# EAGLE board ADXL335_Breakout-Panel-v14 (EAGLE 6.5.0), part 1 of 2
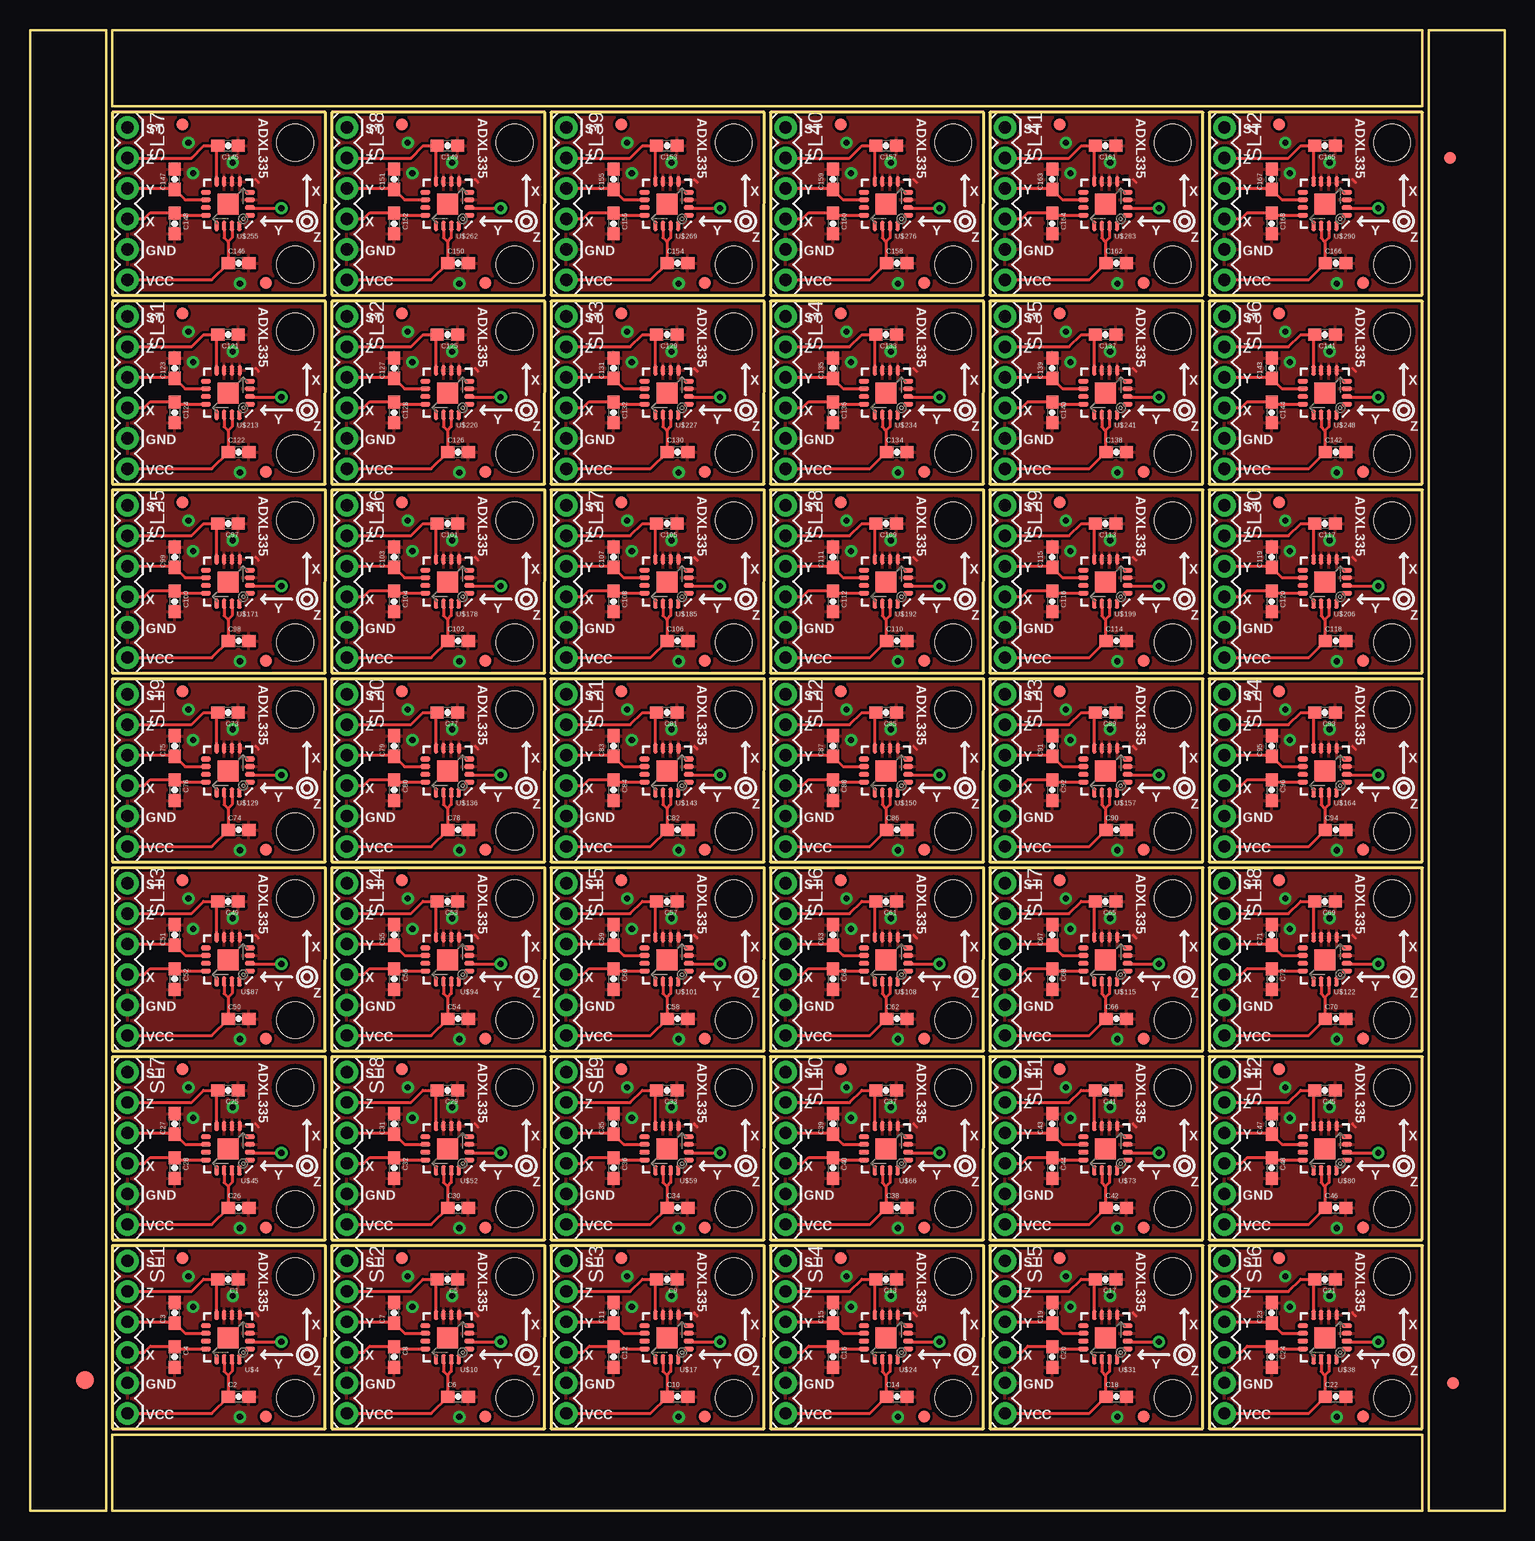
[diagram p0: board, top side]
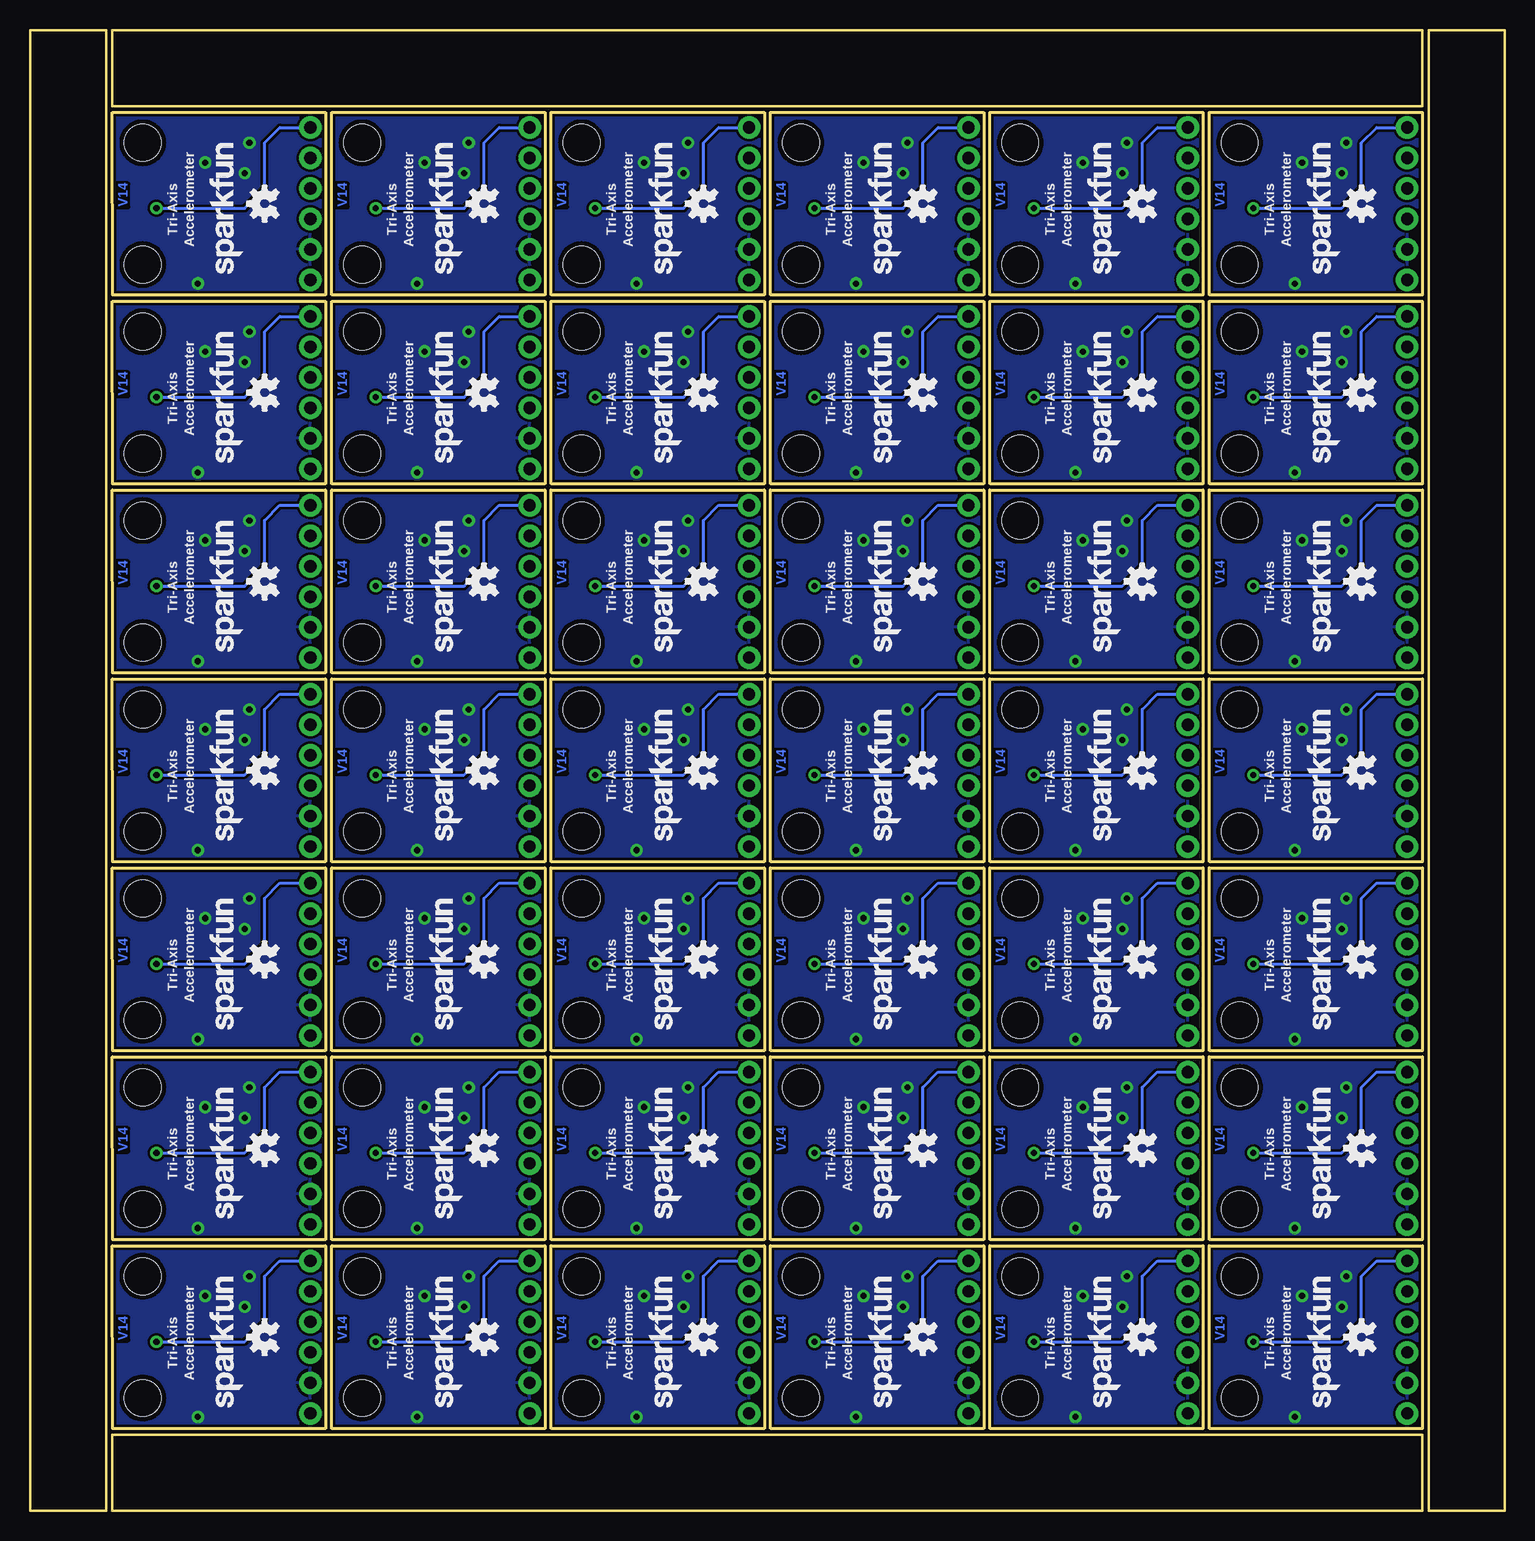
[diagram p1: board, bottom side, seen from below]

Size 122.94 x 123.44 mm. Coordinates in mm from the lower left corner, seen from the top.
Outline: 188 segments
Copper layers (1*16): Top 0.035mm / dielectric 1.5mm / Bottom 0.035mm
Design rules "SparkFun": minimum track width 7mil, minimum drill 15mil, track to track 8mil, track to pad 8mil, pad to pad 8mil, via to via 8mil, smd to smd 8mil, copper to edge 8mil, drill to drill 8mil, minimum pad ring 12mil, minimum via ring 10mil, stop-mask expansion 4mil, vias tented up to drill 20mil, thermal gap 10mil
tRestrict: area 16.4,16.3 to 16.6,16.4; area 17,16.3 to 17.3,16.4; area 18,15.7 to 18.4,16.9; area 34.7,16.3 to 34.9,16.4; area 35.3,16.3 to 35.6,16.4; area 36.3,15.7 to 36.7,16.9; area 53,16.3 to 53.2,16.4; area 53.6,16.3 to 53.9,16.4; area 54.6,15.7 to 55,16.9; area 71.2,16.3 to 71.5,16.4; area 71.9,16.3 to 72.2,16.4; area 72.9,15.7 to 73.3,16.9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

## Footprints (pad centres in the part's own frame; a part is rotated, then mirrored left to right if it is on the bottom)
0603-CAP = smd 1.1 x 1: 1 -0.85,0; 2 0.85,0
FIDUCIAL-1.5X3 = smd 1.5 x 1.5: 1 0,0
FIDUCIAL-1X2 = smd 1 x 1: 1 0,0
1X06 = drill 1.016 pad 1.88: 1 0,0; 2 2.54,0; 3 5.08,0; 4 7.62,0; 5 10.16,0; 6 12.7,0
ADXL335-P = smd 1.75 x 1.75: 0 0,0.051 | smd 0.838 x 0.37: 1 -1.826,0.975; 2 -1.826,0.325; 3 -1.826,-0.325; 4 -1.826,-0.95; 9 1.852,-0.95; 10 1.852,-0.325; 11 1.852,0.325; 12 1.852,0.975 | smd 0.37 x 0.838: 5 -0.975,-1.852; 6 -0.325,-1.852; 7 0.325,-1.852; 8 0.95,-1.852; 13 0.95,1.852; 14 0.325,1.852; 15 -0.325,1.852; 16 -0.95,1.852
STAND-OFF-TIGHT = hole 3.048: 0,0

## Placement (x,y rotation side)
C1  0.1uF  [0603-CAP]  16.51,19.3 180 top
C2  0.1uF  [0603-CAP]  17.4,9.53 0 top
C3  0.1uF  [0603-CAP]  12.06,16.51 90 top
C4  0.1uF  [0603-CAP]  12.06,12.83 270 top
C5  0.1uF  [0603-CAP]  34.8,19.3 180 top
C6  0.1uF  [0603-CAP]  35.69,9.53 0 top
C7  0.1uF  [0603-CAP]  30.35,16.51 90 top
C8  0.1uF  [0603-CAP]  30.35,12.83 270 top
C9  0.1uF  [0603-CAP]  53.09,19.3 180 top
C10  0.1uF  [0603-CAP]  53.98,9.53 0 top
C11  0.1uF  [0603-CAP]  48.64,16.51 90 top
C12  0.1uF  [0603-CAP]  48.64,12.83 270 top
C13  0.1uF  [0603-CAP]  71.37,19.3 180 top
C14  0.1uF  [0603-CAP]  72.26,9.53 0 top
C15  0.1uF  [0603-CAP]  66.93,16.51 90 top
C16  0.1uF  [0603-CAP]  66.93,12.83 270 top
C17  0.1uF  [0603-CAP]  89.66,19.3 180 top
C18  0.1uF  [0603-CAP]  90.55,9.53 0 top
C19  0.1uF  [0603-CAP]  85.22,16.51 90 top
C20  0.1uF  [0603-CAP]  85.22,12.83 270 top
C21  0.1uF  [0603-CAP]  107.95,19.3 180 top
C22  0.1uF  [0603-CAP]  108.84,9.53 0 top
C23  0.1uF  [0603-CAP]  103.5,16.51 90 top
C24  0.1uF  [0603-CAP]  103.5,12.83 270 top
C25  0.1uF  [0603-CAP]  16.51,35.05 180 top
C26  0.1uF  [0603-CAP]  17.4,25.27 0 top
C27  0.1uF  [0603-CAP]  12.06,32.26 90 top
C28  0.1uF  [0603-CAP]  12.06,28.57 270 top
C29  0.1uF  [0603-CAP]  34.8,35.05 180 top
C30  0.1uF  [0603-CAP]  35.69,25.27 0 top
C31  0.1uF  [0603-CAP]  30.35,32.26 90 top
C32  0.1uF  [0603-CAP]  30.35,28.57 270 top
C33  0.1uF  [0603-CAP]  53.09,35.05 180 top
C34  0.1uF  [0603-CAP]  53.98,25.27 0 top
C35  0.1uF  [0603-CAP]  48.64,32.26 90 top
C36  0.1uF  [0603-CAP]  48.64,28.57 270 top
C37  0.1uF  [0603-CAP]  71.37,35.05 180 top
C38  0.1uF  [0603-CAP]  72.26,25.27 0 top
C39  0.1uF  [0603-CAP]  66.93,32.26 90 top
C40  0.1uF  [0603-CAP]  66.93,28.57 270 top
C41  0.1uF  [0603-CAP]  89.66,35.05 180 top
C42  0.1uF  [0603-CAP]  90.55,25.27 0 top
C43  0.1uF  [0603-CAP]  85.22,32.26 90 top
C44  0.1uF  [0603-CAP]  85.22,28.57 270 top
C45  0.1uF  [0603-CAP]  107.95,35.05 180 top
C46  0.1uF  [0603-CAP]  108.84,25.27 0 top
C47  0.1uF  [0603-CAP]  103.5,32.26 90 top
C48  0.1uF  [0603-CAP]  103.5,28.57 270 top
C49  0.1uF  [0603-CAP]  16.51,50.8 180 top
C50  0.1uF  [0603-CAP]  17.4,41.02 0 top
C51  0.1uF  [0603-CAP]  12.06,48.01 90 top
C52  0.1uF  [0603-CAP]  12.06,44.32 270 top
C53  0.1uF  [0603-CAP]  34.8,50.8 180 top
C54  0.1uF  [0603-CAP]  35.69,41.02 0 top
C55  0.1uF  [0603-CAP]  30.35,48.01 90 top
C56  0.1uF  [0603-CAP]  30.35,44.32 270 top
C57  0.1uF  [0603-CAP]  53.09,50.8 180 top
C58  0.1uF  [0603-CAP]  53.98,41.02 0 top
C59  0.1uF  [0603-CAP]  48.64,48.01 90 top
C60  0.1uF  [0603-CAP]  48.64,44.32 270 top
C61  0.1uF  [0603-CAP]  71.37,50.8 180 top
C62  0.1uF  [0603-CAP]  72.26,41.02 0 top
C63  0.1uF  [0603-CAP]  66.93,48.01 90 top
C64  0.1uF  [0603-CAP]  66.93,44.32 270 top
C65  0.1uF  [0603-CAP]  89.66,50.8 180 top
C66  0.1uF  [0603-CAP]  90.55,41.02 0 top
C67  0.1uF  [0603-CAP]  85.22,48.01 90 top
C68  0.1uF  [0603-CAP]  85.22,44.32 270 top
C69  0.1uF  [0603-CAP]  107.95,50.8 180 top
C70  0.1uF  [0603-CAP]  108.84,41.02 0 top
C71  0.1uF  [0603-CAP]  103.5,48.01 90 top
C72  0.1uF  [0603-CAP]  103.5,44.32 270 top
C73  0.1uF  [0603-CAP]  16.51,66.55 180 top
C74  0.1uF  [0603-CAP]  17.4,56.77 0 top
C75  0.1uF  [0603-CAP]  12.06,63.75 90 top
C76  0.1uF  [0603-CAP]  12.06,60.07 270 top
C77  0.1uF  [0603-CAP]  34.8,66.55 180 top
C78  0.1uF  [0603-CAP]  35.69,56.77 0 top
C79  0.1uF  [0603-CAP]  30.35,63.75 90 top
C80  0.1uF  [0603-CAP]  30.35,60.07 270 top
C81  0.1uF  [0603-CAP]  53.09,66.55 180 top
C82  0.1uF  [0603-CAP]  53.98,56.77 0 top
C83  0.1uF  [0603-CAP]  48.64,63.75 90 top
C84  0.1uF  [0603-CAP]  48.64,60.07 270 top
C85  0.1uF  [0603-CAP]  71.37,66.55 180 top
C86  0.1uF  [0603-CAP]  72.26,56.77 0 top
C87  0.1uF  [0603-CAP]  66.93,63.75 90 top
C88  0.1uF  [0603-CAP]  66.93,60.07 270 top
C89  0.1uF  [0603-CAP]  89.66,66.55 180 top
C90  0.1uF  [0603-CAP]  90.55,56.77 0 top
C91  0.1uF  [0603-CAP]  85.22,63.75 90 top
C92  0.1uF  [0603-CAP]  85.22,60.07 270 top
C93  0.1uF  [0603-CAP]  107.95,66.55 180 top
C94  0.1uF  [0603-CAP]  108.84,56.77 0 top
C95  0.1uF  [0603-CAP]  103.5,63.75 90 top
C96  0.1uF  [0603-CAP]  103.5,60.07 270 top
C97  0.1uF  [0603-CAP]  16.51,82.3 180 top
C98  0.1uF  [0603-CAP]  17.4,72.52 0 top
C99  0.1uF  [0603-CAP]  12.06,79.5 90 top
C100  0.1uF  [0603-CAP]  12.06,75.82 270 top
C101  0.1uF  [0603-CAP]  34.8,82.3 180 top
C102  0.1uF  [0603-CAP]  35.69,72.52 0 top
C103  0.1uF  [0603-CAP]  30.35,79.5 90 top
C104  0.1uF  [0603-CAP]  30.35,75.82 270 top
C105  0.1uF  [0603-CAP]  53.09,82.3 180 top
C106  0.1uF  [0603-CAP]  53.98,72.52 0 top
C107  0.1uF  [0603-CAP]  48.64,79.5 90 top
C108  0.1uF  [0603-CAP]  48.64,75.82 270 top
C109  0.1uF  [0603-CAP]  71.37,82.3 180 top
C110  0.1uF  [0603-CAP]  72.26,72.52 0 top
C111  0.1uF  [0603-CAP]  66.93,79.5 90 top
C112  0.1uF  [0603-CAP]  66.93,75.82 270 top
C113  0.1uF  [0603-CAP]  89.66,82.3 180 top
C114  0.1uF  [0603-CAP]  90.55,72.52 0 top
C115  0.1uF  [0603-CAP]  85.22,79.5 90 top
C116  0.1uF  [0603-CAP]  85.22,75.82 270 top
C117  0.1uF  [0603-CAP]  107.95,82.3 180 top
C118  0.1uF  [0603-CAP]  108.84,72.52 0 top
C119  0.1uF  [0603-CAP]  103.5,79.5 90 top
C120  0.1uF  [0603-CAP]  103.5,75.82 270 top
C121  0.1uF  [0603-CAP]  16.51,98.04 180 top
C122  0.1uF  [0603-CAP]  17.4,88.27 0 top
C123  0.1uF  [0603-CAP]  12.06,95.25 90 top
C124  0.1uF  [0603-CAP]  12.06,91.57 270 top
C125  0.1uF  [0603-CAP]  34.8,98.04 180 top
C126  0.1uF  [0603-CAP]  35.69,88.27 0 top
C127  0.1uF  [0603-CAP]  30.35,95.25 90 top
C128  0.1uF  [0603-CAP]  30.35,91.57 270 top
C129  0.1uF  [0603-CAP]  53.09,98.04 180 top
C130  0.1uF  [0603-CAP]  53.98,88.27 0 top
C131  0.1uF  [0603-CAP]  48.64,95.25 90 top
C132  0.1uF  [0603-CAP]  48.64,91.57 270 top
C133  0.1uF  [0603-CAP]  71.37,98.04 180 top
C134  0.1uF  [0603-CAP]  72.26,88.27 0 top
C135  0.1uF  [0603-CAP]  66.93,95.25 90 top
C136  0.1uF  [0603-CAP]  66.93,91.57 270 top
C137  0.1uF  [0603-CAP]  89.66,98.04 180 top
C138  0.1uF  [0603-CAP]  90.55,88.27 0 top
C139  0.1uF  [0603-CAP]  85.22,95.25 90 top
C140  0.1uF  [0603-CAP]  85.22,91.57 270 top
C141  0.1uF  [0603-CAP]  107.95,98.04 180 top
C142  0.1uF  [0603-CAP]  108.84,88.27 0 top
C143  0.1uF  [0603-CAP]  103.5,95.25 90 top
C144  0.1uF  [0603-CAP]  103.5,91.57 270 top
C145  0.1uF  [0603-CAP]  16.51,113.79 180 top
C146  0.1uF  [0603-CAP]  17.4,104.01 0 top
C147  0.1uF  [0603-CAP]  12.06,111 90 top
C148  0.1uF  [0603-CAP]  12.06,107.31 270 top
C149  0.1uF  [0603-CAP]  34.8,113.79 180 top
C150  0.1uF  [0603-CAP]  35.69,104.01 0 top
C151  0.1uF  [0603-CAP]  30.35,111 90 top
C152  0.1uF  [0603-CAP]  30.35,107.31 270 top
C153  0.1uF  [0603-CAP]  53.09,113.79 180 top
C154  0.1uF  [0603-CAP]  53.98,104.01 0 top
C155  0.1uF  [0603-CAP]  48.64,111 90 top
C156  0.1uF  [0603-CAP]  48.64,107.31 270 top
C157  0.1uF  [0603-CAP]  71.37,113.79 180 top
C158  0.1uF  [0603-CAP]  72.26,104.01 0 top
C159  0.1uF  [0603-CAP]  66.93,111 90 top
C160  0.1uF  [0603-CAP]  66.93,107.31 270 top
C161  0.1uF  [0603-CAP]  89.66,113.79 180 top
C162  0.1uF  [0603-CAP]  90.55,104.01 0 top
C163  0.1uF  [0603-CAP]  85.22,111 90 top
C164  0.1uF  [0603-CAP]  85.22,107.31 270 top
C165  0.1uF  [0603-CAP]  107.95,113.79 180 top
C166  0.1uF  [0603-CAP]  108.84,104.01 0 top
C167  0.1uF  [0603-CAP]  103.5,111 90 top
C168  0.1uF  [0603-CAP]  103.5,107.31 270 top
E$1  [FIDUCIAL-1.5X3]  4.57,10.92 0 top
E$4  [FIDUCIAL-1X2]  118.62,10.67 0 top
E$5  [FIDUCIAL-1X2]  118.36,112.78 180 top
SL1  [1X06]  8.13,20.83 270 top
SL2  [1X06]  26.42,20.83 270 top
SL3  [1X06]  44.7,20.83 270 top
SL4  [1X06]  62.99,20.83 270 top
SL5  [1X06]  81.28,20.83 270 top
SL6  [1X06]  99.57,20.83 270 top
SL7  [1X06]  8.13,36.58 270 top
SL8  [1X06]  26.42,36.58 270 top
SL9  [1X06]  44.7,36.58 270 top
SL10  [1X06]  62.99,36.58 270 top
SL11  [1X06]  81.28,36.58 270 top
SL12  [1X06]  99.57,36.58 270 top
SL13  [1X06]  8.13,52.32 270 top
SL14  [1X06]  26.42,52.32 270 top
SL15  [1X06]  44.7,52.32 270 top
SL16  [1X06]  62.99,52.32 270 top
SL17  [1X06]  81.28,52.32 270 top
SL18  [1X06]  99.57,52.32 270 top
SL19  [1X06]  8.13,68.07 270 top
SL20  [1X06]  26.42,68.07 270 top
SL21  [1X06]  44.7,68.07 270 top
SL22  [1X06]  62.99,68.07 270 top
SL23  [1X06]  81.28,68.07 270 top
SL24  [1X06]  99.57,68.07 270 top
SL25  [1X06]  8.13,83.82 270 top
SL26  [1X06]  26.42,83.82 270 top
SL27  [1X06]  44.7,83.82 270 top
SL28  [1X06]  62.99,83.82 270 top
SL29  [1X06]  81.28,83.82 270 top
SL30  [1X06]  99.57,83.82 270 top
SL31  [1X06]  8.13,99.57 270 top
SL32  [1X06]  26.42,99.57 270 top
SL33  [1X06]  44.7,99.57 270 top
SL34  [1X06]  62.99,99.57 270 top
SL35  [1X06]  81.28,99.57 270 top
SL36  [1X06]  99.57,99.57 270 top
SL37  [1X06]  8.13,115.32 270 top
SL38  [1X06]  26.42,115.32 270 top
SL39  [1X06]  44.7,115.32 270 top
SL40  [1X06]  62.99,115.32 270 top
SL41  [1X06]  81.28,115.32 270 top
SL42  [1X06]  99.57,115.32 270 top
U$1  FIDUCIAL1X2  [FIDUCIAL-1X2]  12.7,21.08 0 top
U$2  FIDUCIAL1X2  [FIDUCIAL-1X2]  30.99,21.08 0 top
U$3  FIDUCIAL1X2  [FIDUCIAL-1X2]  19.68,7.87 0 top
U$4  ADXL335-PATRICK""  [ADXL335-P]  16.51,14.48 180 top
U$5  [OSHW-LOGO-S]  11.94,14.48 90 bottom
U$6  [STAND-OFF-TIGHT]  22.1,9.4 0 top
U$7  [STAND-OFF-TIGHT]  22.1,19.56 0 top
U$8  [SFE_LOGO_NAME_.1]  13.21,8.13 90 bottom
U$9  FIDUCIAL1X2  [FIDUCIAL-1X2]  37.97,7.87 0 top
U$10  ADXL335-PATRICK""  [ADXL335-P]  34.8,14.48 180 top
U$11  [STAND-OFF-TIGHT]  40.39,9.4 0 top
U$12  [STAND-OFF-TIGHT]  40.39,19.56 0 top
U$13  [OSHW-LOGO-S]  30.23,14.48 90 bottom
U$14  [SFE_LOGO_NAME_.1]  31.5,8.13 90 bottom
U$15  FIDUCIAL1X2  [FIDUCIAL-1X2]  49.28,21.08 0 top
U$16  FIDUCIAL1X2  [FIDUCIAL-1X2]  56.26,7.87 0 top
U$17  ADXL335-PATRICK""  [ADXL335-P]  53.09,14.48 180 top
U$18  [STAND-OFF-TIGHT]  58.67,9.4 0 top
U$19  [STAND-OFF-TIGHT]  58.67,19.56 0 top
U$20  [OSHW-LOGO-S]  48.51,14.48 90 bottom
U$21  [SFE_LOGO_NAME_.1]  49.78,8.13 90 bottom
U$22  FIDUCIAL1X2  [FIDUCIAL-1X2]  67.56,21.08 0 top
U$23  FIDUCIAL1X2  [FIDUCIAL-1X2]  74.55,7.87 0 top
U$24  ADXL335-PATRICK""  [ADXL335-P]  71.37,14.48 180 top
U$25  [STAND-OFF-TIGHT]  76.96,9.4 0 top
U$26  [STAND-OFF-TIGHT]  76.96,19.56 0 top
U$27  [OSHW-LOGO-S]  66.8,14.48 90 bottom
U$28  [SFE_LOGO_NAME_.1]  68.07,8.13 90 bottom
U$29  FIDUCIAL1X2  [FIDUCIAL-1X2]  85.85,21.08 0 top
U$30  FIDUCIAL1X2  [FIDUCIAL-1X2]  92.84,7.87 0 top
U$31  ADXL335-PATRICK""  [ADXL335-P]  89.66,14.48 180 top
U$32  [STAND-OFF-TIGHT]  95.25,9.4 0 top
U$33  [STAND-OFF-TIGHT]  95.25,19.56 0 top
U$34  [OSHW-LOGO-S]  85.09,14.48 90 bottom
U$35  [SFE_LOGO_NAME_.1]  86.36,8.13 90 bottom
U$36  FIDUCIAL1X2  [FIDUCIAL-1X2]  104.14,21.08 0 top
U$37  FIDUCIAL1X2  [FIDUCIAL-1X2]  111.12,7.87 0 top
U$38  ADXL335-PATRICK""  [ADXL335-P]  107.95,14.48 180 top
U$39  [STAND-OFF-TIGHT]  113.54,9.4 0 top
U$40  [STAND-OFF-TIGHT]  113.54,19.56 0 top
U$41  [OSHW-LOGO-S]  103.38,14.48 90 bottom
U$42  [SFE_LOGO_NAME_.1]  104.65,8.13 90 bottom
U$43  FIDUCIAL1X2  [FIDUCIAL-1X2]  12.7,36.83 0 top
U$44  FIDUCIAL1X2  [FIDUCIAL-1X2]  19.68,23.62 0 top
U$45  ADXL335-PATRICK""  [ADXL335-P]  16.51,30.23 180 top
U$46  [STAND-OFF-TIGHT]  22.1,25.15 0 top
U$47  [STAND-OFF-TIGHT]  22.1,35.31 0 top
U$48  [OSHW-LOGO-S]  11.94,30.23 90 bottom
U$49  [SFE_LOGO_NAME_.1]  13.21,23.88 90 bottom
U$50  FIDUCIAL1X2  [FIDUCIAL-1X2]  30.99,36.83 0 top
U$51  FIDUCIAL1X2  [FIDUCIAL-1X2]  37.97,23.62 0 top
U$52  ADXL335-PATRICK""  [ADXL335-P]  34.8,30.23 180 top
U$53  [STAND-OFF-TIGHT]  40.39,25.15 0 top
U$54  [STAND-OFF-TIGHT]  40.39,35.31 0 top
U$55  [OSHW-LOGO-S]  30.23,30.23 90 bottom
U$56  [SFE_LOGO_NAME_.1]  31.5,23.88 90 bottom
U$57  FIDUCIAL1X2  [FIDUCIAL-1X2]  49.28,36.83 0 top
U$58  FIDUCIAL1X2  [FIDUCIAL-1X2]  56.26,23.62 0 top
U$59  ADXL335-PATRICK""  [ADXL335-P]  53.09,30.23 180 top
U$60  [STAND-OFF-TIGHT]  58.67,25.15 0 top
U$61  [STAND-OFF-TIGHT]  58.67,35.31 0 top
U$62  [OSHW-LOGO-S]  48.51,30.23 90 bottom
U$63  [SFE_LOGO_NAME_.1]  49.78,23.88 90 bottom
U$64  FIDUCIAL1X2  [FIDUCIAL-1X2]  67.56,36.83 0 top
U$65  FIDUCIAL1X2  [FIDUCIAL-1X2]  74.55,23.62 0 top
U$66  ADXL335-PATRICK""  [ADXL335-P]  71.37,30.23 180 top
U$67  [STAND-OFF-TIGHT]  76.96,25.15 0 top
U$68  [STAND-OFF-TIGHT]  76.96,35.31 0 top
U$69  [OSHW-LOGO-S]  66.8,30.23 90 bottom
U$70  [SFE_LOGO_NAME_.1]  68.07,23.88 90 bottom
U$71  FIDUCIAL1X2  [FIDUCIAL-1X2]  85.85,36.83 0 top
U$72  FIDUCIAL1X2  [FIDUCIAL-1X2]  92.84,23.62 0 top
U$73  ADXL335-PATRICK""  [ADXL335-P]  89.66,30.23 180 top
U$74  [STAND-OFF-TIGHT]  95.25,25.15 0 top
U$75  [STAND-OFF-TIGHT]  95.25,35.31 0 top
U$76  [OSHW-LOGO-S]  85.09,30.23 90 bottom
U$77  [SFE_LOGO_NAME_.1]  86.36,23.88 90 bottom
U$78  FIDUCIAL1X2  [FIDUCIAL-1X2]  104.14,36.83 0 top
U$79  FIDUCIAL1X2  [FIDUCIAL-1X2]  111.12,23.62 0 top
U$80  ADXL335-PATRICK""  [ADXL335-P]  107.95,30.23 180 top
U$81  [STAND-OFF-TIGHT]  113.54,25.15 0 top
U$82  [STAND-OFF-TIGHT]  113.54,35.31 0 top
U$83  [OSHW-LOGO-S]  103.38,30.23 90 bottom
U$84  [SFE_LOGO_NAME_.1]  104.65,23.88 90 bottom
U$85  FIDUCIAL1X2  [FIDUCIAL-1X2]  12.7,52.58 0 top
U$86  FIDUCIAL1X2  [FIDUCIAL-1X2]  19.68,39.37 0 top
U$87  ADXL335-PATRICK""  [ADXL335-P]  16.51,45.97 180 top
U$88  [STAND-OFF-TIGHT]  22.1,40.89 0 top
U$89  [STAND-OFF-TIGHT]  22.1,51.05 0 top
U$90  [OSHW-LOGO-S]  11.94,45.97 90 bottom
U$91  [SFE_LOGO_NAME_.1]  13.21,39.62 90 bottom
U$92  FIDUCIAL1X2  [FIDUCIAL-1X2]  30.99,52.58 0 top
U$93  FIDUCIAL1X2  [FIDUCIAL-1X2]  37.97,39.37 0 top
U$94  ADXL335-PATRICK""  [ADXL335-P]  34.8,45.97 180 top
U$95  [STAND-OFF-TIGHT]  40.39,40.89 0 top
U$96  [STAND-OFF-TIGHT]  40.39,51.05 0 top
U$97  [OSHW-LOGO-S]  30.23,45.97 90 bottom
U$98  [SFE_LOGO_NAME_.1]  31.5,39.62 90 bottom
U$99  FIDUCIAL1X2  [FIDUCIAL-1X2]  49.28,52.58 0 top
U$100  FIDUCIAL1X2  [FIDUCIAL-1X2]  56.26,39.37 0 top
U$101  ADXL335-PATRICK""  [ADXL335-P]  53.09,45.97 180 top
U$102  [STAND-OFF-TIGHT]  58.67,40.89 0 top
U$103  [STAND-OFF-TIGHT]  58.67,51.05 0 top
U$104  [OSHW-LOGO-S]  48.51,45.97 90 bottom
U$105  [SFE_LOGO_NAME_.1]  49.78,39.62 90 bottom
U$106  FIDUCIAL1X2  [FIDUCIAL-1X2]  67.56,52.58 0 top
U$107  FIDUCIAL1X2  [FIDUCIAL-1X2]  74.55,39.37 0 top
U$108  ADXL335-PATRICK""  [ADXL335-P]  71.37,45.97 180 top
U$109  [STAND-OFF-TIGHT]  76.96,40.89 0 top
U$110  [STAND-OFF-TIGHT]  76.96,51.05 0 top
U$111  [OSHW-LOGO-S]  66.8,45.97 90 bottom
U$112  [SFE_LOGO_NAME_.1]  68.07,39.62 90 bottom
U$113  FIDUCIAL1X2  [FIDUCIAL-1X2]  85.85,52.58 0 top
U$114  FIDUCIAL1X2  [FIDUCIAL-1X2]  92.84,39.37 0 top
U$115  ADXL335-PATRICK""  [ADXL335-P]  89.66,45.97 180 top
U$116  [STAND-OFF-TIGHT]  95.25,40.89 0 top
U$117  [STAND-OFF-TIGHT]  95.25,51.05 0 top
U$118  [OSHW-LOGO-S]  85.09,45.97 90 bottom
U$119  [SFE_LOGO_NAME_.1]  86.36,39.62 90 bottom
U$120  FIDUCIAL1X2  [FIDUCIAL-1X2]  104.14,52.58 0 top
U$121  FIDUCIAL1X2  [FIDUCIAL-1X2]  111.12,39.37 0 top
U$122  ADXL335-PATRICK""  [ADXL335-P]  107.95,45.97 180 top
U$123  [STAND-OFF-TIGHT]  113.54,40.89 0 top
U$124  [STAND-OFF-TIGHT]  113.54,51.05 0 top
U$125  [OSHW-LOGO-S]  103.38,45.97 90 bottom
U$126  [SFE_LOGO_NAME_.1]  104.65,39.62 90 bottom
U$127  FIDUCIAL1X2  [FIDUCIAL-1X2]  12.7,68.33 0 top
U$128  FIDUCIAL1X2  [FIDUCIAL-1X2]  19.68,55.12 0 top
U$129  ADXL335-PATRICK""  [ADXL335-P]  16.51,61.72 180 top
U$130  [STAND-OFF-TIGHT]  22.1,56.64 0 top
U$131  [STAND-OFF-TIGHT]  22.1,66.8 0 top
U$132  [OSHW-LOGO-S]  11.94,61.72 90 bottom
U$133  [SFE_LOGO_NAME_.1]  13.21,55.37 90 bottom
U$134  FIDUCIAL1X2  [FIDUCIAL-1X2]  30.99,68.33 0 top
U$135  FIDUCIAL1X2  [FIDUCIAL-1X2]  37.97,55.12 0 top
U$136  ADXL335-PATRICK""  [ADXL335-P]  34.8,61.72 180 top
U$137  [STAND-OFF-TIGHT]  40.39,56.64 0 top
U$138  [STAND-OFF-TIGHT]  40.39,66.8 0 top
U$139  [OSHW-LOGO-S]  30.23,61.72 90 bottom
U$140  [SFE_LOGO_NAME_.1]  31.5,55.37 90 bottom
U$141  FIDUCIAL1X2  [FIDUCIAL-1X2]  49.28,68.33 0 top
U$142  FIDUCIAL1X2  [FIDUCIAL-1X2]  56.26,55.12 0 top
U$143  ADXL335-PATRICK""  [ADXL335-P]  53.09,61.72 180 top
U$144  [STAND-OFF-TIGHT]  58.67,56.64 0 top
U$145  [STAND-OFF-TIGHT]  58.67,66.8 0 top
U$146  [OSHW-LOGO-S]  48.51,61.72 90 bottom
U$147  [SFE_LOGO_NAME_.1]  49.78,55.37 90 bottom
U$148  FIDUCIAL1X2  [FIDUCIAL-1X2]  67.56,68.33 0 top
U$149  FIDUCIAL1X2  [FIDUCIAL-1X2]  74.55,55.12 0 top
U$150  ADXL335-PATRICK""  [ADXL335-P]  71.37,61.72 180 top
U$151  [STAND-OFF-TIGHT]  76.96,56.64 0 top
U$152  [STAND-OFF-TIGHT]  76.96,66.8 0 top
U$153  [OSHW-LOGO-S]  66.8,61.72 90 bottom
U$154  [SFE_LOGO_NAME_.1]  68.07,55.37 90 bottom
U$155  FIDUCIAL1X2  [FIDUCIAL-1X2]  85.85,68.33 0 top
U$156  FIDUCIAL1X2  [FIDUCIAL-1X2]  92.84,55.12 0 top
U$157  ADXL335-PATRICK""  [ADXL335-P]  89.66,61.72 180 top
U$158  [STAND-OFF-TIGHT]  95.25,56.64 0 top
U$159  [STAND-OFF-TIGHT]  95.25,66.8 0 top
U$160  [OSHW-LOGO-S]  85.09,61.72 90 bottom
U$161  [SFE_LOGO_NAME_.1]  86.36,55.37 90 bottom
U$162  FIDUCIAL1X2  [FIDUCIAL-1X2]  104.14,68.33 0 top
U$163  FIDUCIAL1X2  [FIDUCIAL-1X2]  111.12,55.12 0 top
U$164  ADXL335-PATRICK""  [ADXL335-P]  107.95,61.72 180 top
U$165  [STAND-OFF-TIGHT]  113.54,56.64 0 top
U$166  [STAND-OFF-TIGHT]  113.54,66.8 0 top
U$167  [OSHW-LOGO-S]  103.38,61.72 90 bottom
U$168  [SFE_LOGO_NAME_.1]  104.65,55.37 90 bottom
U$169  FIDUCIAL1X2  [FIDUCIAL-1X2]  12.7,84.07 0 top
U$170  FIDUCIAL1X2  [FIDUCIAL-1X2]  19.68,70.87 0 top
U$171  ADXL335-PATRICK""  [ADXL335-P]  16.51,77.47 180 top
U$172  [STAND-OFF-TIGHT]  22.1,72.39 0 top
U$173  [STAND-OFF-TIGHT]  22.1,82.55 0 top
U$174  [OSHW-LOGO-S]  11.94,77.47 90 bottom
U$175  [SFE_LOGO_NAME_.1]  13.21,71.12 90 bottom
U$176  FIDUCIAL1X2  [FIDUCIAL-1X2]  30.99,84.07 0 top
U$177  FIDUCIAL1X2  [FIDUCIAL-1X2]  37.97,70.87 0 top
U$178  ADXL335-PATRICK""  [ADXL335-P]  34.8,77.47 180 top
U$179  [STAND-OFF-TIGHT]  40.39,72.39 0 top
U$180  [STAND-OFF-TIGHT]  40.39,82.55 0 top
U$181  [OSHW-LOGO-S]  30.23,77.47 90 bottom
U$182  [SFE_LOGO_NAME_.1]  31.5,71.12 90 bottom
U$183  FIDUCIAL1X2  [FIDUCIAL-1X2]  49.28,84.07 0 top
U$184  FIDUCIAL1X2  [FIDUCIAL-1X2]  56.26,70.87 0 top
U$185  ADXL335-PATRICK""  [ADXL335-P]  53.09,77.47 180 top
U$186  [STAND-OFF-TIGHT]  58.67,72.39 0 top
U$187  [STAND-OFF-TIGHT]  58.67,82.55 0 top
U$188  [OSHW-LOGO-S]  48.51,77.47 90 bottom
U$189  [SFE_LOGO_NAME_.1]  49.78,71.12 90 bottom
U$190  FIDUCIAL1X2  [FIDUCIAL-1X2]  67.56,84.07 0 top
U$191  FIDUCIAL1X2  [FIDUCIAL-1X2]  74.55,70.87 0 top
U$192  ADXL335-PATRICK""  [ADXL335-P]  71.37,77.47 180 top
U$193  [STAND-OFF-TIGHT]  76.96,72.39 0 top
U$194  [STAND-OFF-TIGHT]  76.96,82.55 0 top
U$195  [OSHW-LOGO-S]  66.8,77.47 90 bottom
U$196  [SFE_LOGO_NAME_.1]  68.07,71.12 90 bottom
U$197  FIDUCIAL1X2  [FIDUCIAL-1X2]  85.85,84.07 0 top
U$198  FIDUCIAL1X2  [FIDUCIAL-1X2]  92.84,70.87 0 top
U$199  ADXL335-PATRICK""  [ADXL335-P]  89.66,77.47 180 top
U$200  [STAND-OFF-TIGHT]  95.25,72.39 0 top
U$201  [STAND-OFF-TIGHT]  95.25,82.55 0 top
U$202  [OSHW-LOGO-S]  85.09,77.47 90 bottom
U$203  [SFE_LOGO_NAME_.1]  86.36,71.12 90 bottom
U$204  FIDUCIAL1X2  [FIDUCIAL-1X2]  104.14,84.07 0 top
U$205  FIDUCIAL1X2  [FIDUCIAL-1X2]  111.12,70.87 0 top
U$206  ADXL335-PATRICK""  [ADXL335-P]  107.95,77.47 180 top
U$207  [STAND-OFF-TIGHT]  113.54,72.39 0 top
U$208  [STAND-OFF-TIGHT]  113.54,82.55 0 top
U$209  [OSHW-LOGO-S]  103.38,77.47 90 bottom
U$210  [SFE_LOGO_NAME_.1]  104.65,71.12 90 bottom
U$211  FIDUCIAL1X2  [FIDUCIAL-1X2]  12.7,99.82 0 top
U$212  FIDUCIAL1X2  [FIDUCIAL-1X2]  19.68,86.61 0 top
U$213  ADXL335-PATRICK""  [ADXL335-P]  16.51,93.22 180 top
U$214  [STAND-OFF-TIGHT]  22.1,88.14 0 top
U$215  [STAND-OFF-TIGHT]  22.1,98.3 0 top
U$216  [OSHW-LOGO-S]  11.94,93.22 90 bottom
U$217  [SFE_LOGO_NAME_.1]  13.21,86.87 90 bottom
U$218  FIDUCIAL1X2  [FIDUCIAL-1X2]  30.99,99.82 0 top
U$219  FIDUCIAL1X2  [FIDUCIAL-1X2]  37.97,86.61 0 top
U$220  ADXL335-PATRICK""  [ADXL335-P]  34.8,93.22 180 top
U$221  [STAND-OFF-TIGHT]  40.39,88.14 0 top
U$222  [STAND-OFF-TIGHT]  40.39,98.3 0 top
U$223  [OSHW-LOGO-S]  30.23,93.22 90 bottom
U$224  [SFE_LOGO_NAME_.1]  31.5,86.87 90 bottom
U$225  FIDUCIAL1X2  [FIDUCIAL-1X2]  49.28,99.82 0 top
U$226  FIDUCIAL1X2  [FIDUCIAL-1X2]  56.26,86.61 0 top
U$227  ADXL335-PATRICK""  [ADXL335-P]  53.09,93.22 180 top
U$228  [STAND-OFF-TIGHT]  58.67,88.14 0 top
U$229  [STAND-OFF-TIGHT]  58.67,98.3 0 top
U$230  [OSHW-LOGO-S]  48.51,93.22 90 bottom
U$231  [SFE_LOGO_NAME_.1]  49.78,86.87 90 bottom
U$232  FIDUCIAL1X2  [FIDUCIAL-1X2]  67.56,99.82 0 top
U$233  FIDUCIAL1X2  [FIDUCIAL-1X2]  74.55,86.61 0 top
U$234  ADXL335-PATRICK""  [ADXL335-P]  71.37,93.22 180 top
U$235  [STAND-OFF-TIGHT]  76.96,88.14 0 top
U$236  [STAND-OFF-TIGHT]  76.96,98.3 0 top
U$237  [OSHW-LOGO-S]  66.8,93.22 90 bottom
U$238  [SFE_LOGO_NAME_.1]  68.07,86.87 90 bottom
U$239  FIDUCIAL1X2  [FIDUCIAL-1X2]  85.85,99.82 0 top
U$240  FIDUCIAL1X2  [FIDUCIAL-1X2]  92.84,86.61 0 top
U$241  ADXL335-PATRICK""  [ADXL335-P]  89.66,93.22 180 top
U$242  [STAND-OFF-TIGHT]  95.25,88.14 0 top
U$243  [STAND-OFF-TIGHT]  95.25,98.3 0 top
U$244  [OSHW-LOGO-S]  85.09,93.22 90 bottom
U$245  [SFE_LOGO_NAME_.1]  86.36,86.87 90 bottom
U$246  FIDUCIAL1X2  [FIDUCIAL-1X2]  104.14,99.82 0 top
U$247  FIDUCIAL1X2  [FIDUCIAL-1X2]  111.12,86.61 0 top
U$248  ADXL335-PATRICK""  [ADXL335-P]  107.95,93.22 180 top
U$249  [STAND-OFF-TIGHT]  113.54,88.14 0 top
U$250  [STAND-OFF-TIGHT]  113.54,98.3 0 top
U$251  [OSHW-LOGO-S]  103.38,93.22 90 bottom
U$252  [SFE_LOGO_NAME_.1]  104.65,86.87 90 bottom
U$253  FIDUCIAL1X2  [FIDUCIAL-1X2]  12.7,115.57 0 top
U$254  FIDUCIAL1X2  [FIDUCIAL-1X2]  19.68,102.36 0 top
U$255  ADXL335-PATRICK""  [ADXL335-P]  16.51,108.97 180 top
U$256  [STAND-OFF-TIGHT]  22.1,103.89 0 top
U$257  [STAND-OFF-TIGHT]  22.1,114.05 0 top
U$258  [OSHW-LOGO-S]  11.94,108.97 90 bottom
U$259  [SFE_LOGO_NAME_.1]  13.21,102.62 90 bottom
U$260  FIDUCIAL1X2  [FIDUCIAL-1X2]  30.99,115.57 0 top
U$261  FIDUCIAL1X2  [FIDUCIAL-1X2]  37.97,102.36 0 top
U$262  ADXL335-PATRICK""  [ADXL335-P]  34.8,108.97 180 top
U$263  [STAND-OFF-TIGHT]  40.39,103.89 0 top
U$264  [STAND-OFF-TIGHT]  40.39,114.05 0 top
U$265  [OSHW-LOGO-S]  30.23,108.97 90 bottom
U$266  [SFE_LOGO_NAME_.1]  31.5,102.62 90 bottom
U$267  FIDUCIAL1X2  [FIDUCIAL-1X2]  49.28,115.57 0 top
U$268  FIDUCIAL1X2  [FIDUCIAL-1X2]  56.26,102.36 0 top
U$269  ADXL335-PATRICK""  [ADXL335-P]  53.09,108.97 180 top
U$270  [STAND-OFF-TIGHT]  58.67,103.89 0 top
U$271  [STAND-OFF-TIGHT]  58.67,114.05 0 top
U$272  [OSHW-LOGO-S]  48.51,108.97 90 bottom
U$273  [SFE_LOGO_NAME_.1]  49.78,102.62 90 bottom
U$274  FIDUCIAL1X2  [FIDUCIAL-1X2]  67.56,115.57 0 top
U$275  FIDUCIAL1X2  [FIDUCIAL-1X2]  74.55,102.36 0 top
U$276  ADXL335-PATRICK""  [ADXL335-P]  71.37,108.97 180 top
U$277  [STAND-OFF-TIGHT]  76.96,103.89 0 top
U$278  [STAND-OFF-TIGHT]  76.96,114.05 0 top
U$279  [OSHW-LOGO-S]  66.8,108.97 90 bottom
U$280  [SFE_LOGO_NAME_.1]  68.07,102.62 90 bottom
U$281  FIDUCIAL1X2  [FIDUCIAL-1X2]  85.85,115.57 0 top
U$282  FIDUCIAL1X2  [FIDUCIAL-1X2]  92.84,102.36 0 top
U$283  ADXL335-PATRICK""  [ADXL335-P]  89.66,108.97 180 top
U$284  [STAND-OFF-TIGHT]  95.25,103.89 0 top
U$285  [STAND-OFF-TIGHT]  95.25,114.05 0 top
U$286  [OSHW-LOGO-S]  85.09,108.97 90 bottom
U$287  [SFE_LOGO_NAME_.1]  86.36,102.62 90 bottom
U$288  FIDUCIAL1X2  [FIDUCIAL-1X2]  104.14,115.57 0 top
U$289  FIDUCIAL1X2  [FIDUCIAL-1X2]  111.12,102.36 0 top
U$290  ADXL335-PATRICK""  [ADXL335-P]  107.95,108.97 180 top
U$291  [STAND-OFF-TIGHT]  113.54,103.89 0 top
U$292  [STAND-OFF-TIGHT]  113.54,114.05 0 top
U$293  [OSHW-LOGO-S]  103.38,108.97 90 bottom
U$294  [SFE_LOGO_NAME_.1]  104.65,102.62 90 bottom

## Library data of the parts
C1-C168 SL1-SL42 U$1-U$3 U$6 U$7 U$9 U$11 U$12 U$15 U$16 U$18 U$19 U$22 U$23 U$25 U$26 U$29 U$30 U$32 U$33 U$36 U$37 U$39 U$40 U$43 U$44 U$46 U$47 U$50 U$51 U$53 U$54 U$57 U$58 U$60 U$61 U$64 U$65 U$67 U$68 U$71 U$72 U$74 U$75 U$78 U$79 U$81 U$82 U$85 U$86 U$88 U$89 U$92 U$93 U$95 U$96 U$99 U$100 U$102 U$103 U$106 U$107 U$109 U$110 U$113 U$114 U$116 U$117 U$120 U$121 U$123 U$124 U$127 U$128 U$130 U$131 U$134 U$135 U$137 U$138 U$141 U$142 U$144 U$145 U$148 U$149 U$151 U$152 U$155 U$156 U$158 U$159 U$162 U$163 U$165 U$166 U$169 U$170 U$172 U$173 U$176 U$177 U$179 U$180 U$183 U$184 U$186 U$187 U$190 U$191 U$193 U$194 U$197 U$198 U$200 U$201 U$204 U$205 U$207 U$208 U$211 U$212 U$214 U$215 U$218 U$219 U$221 U$222 U$225 U$226 U$228 U$229 U$232 U$233 U$235 U$236 U$239 U$240 U$242 U$243 U$246 U$247 U$249 U$250 U$253 U$254 U$256 U$257 U$260 U$261 U$263 U$264 U$267 U$268 U$270 U$271 U$274 U$275 U$277 U$278 U$281 U$282 U$284 U$285 U$288 U$289 U$291 U$292 = SparkFun
E$1 E$4 E$5 U$5 U$8 U$13 U$14 U$20 U$21 U$27 U$28 U$34 U$35 U$41 U$42 U$48 U$49 U$55 U$56 U$62 U$63 U$69 U$70 U$76 U$77 U$83 U$84 U$90 U$91 U$97 U$98 U$104 U$105 U$111 U$112 U$118 U$119 U$125 U$126 U$132 U$133 U$139 U$140 U$146 U$147 U$153 U$154 U$160 U$161 U$167 U$168 U$174 U$175 U$181 U$182 U$188 U$189 U$195 U$196 U$202 U$203 U$209 U$210 U$216 U$217 U$223 U$224 U$230 U$231 U$237 U$238 U$244 U$245 U$251 U$252 U$258 U$259 U$265 U$266 U$272 U$273 U$279 U$280 U$286 U$287 U$293 U$294 = SparkFun-Aesthetics
U$4 U$10 U$17 U$24 U$31 U$38 U$45 U$52 U$59 U$66 U$73 U$80 U$87 U$94 U$101 U$108 U$115 U$122 U$129 U$136 U$143 U$150 U$157 U$164 U$171 U$178 U$185 U$192 U$199 U$206 U$213 U$220 U$227 U$234 U$241 U$248 U$255 U$262 U$269 U$276 U$283 U$290 = Testing

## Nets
GND: C1.1 C2.2 C3.2 C4.2 SL1.5 U$4.3 U$4.5 U$4.6 U$4.7
GND1: C5.1 C6.2 C7.2 C8.2 SL2.5 U$10.3 U$10.5 U$10.6 U$10.7
GND2: C9.1 C10.2 C11.2 C12.2 SL3.5 U$17.3 U$17.5 U$17.6 U$17.7
GND3: C13.1 C14.2 C15.2 C16.2 SL4.5 U$24.3 U$24.5 U$24.6 U$24.7
GND4: C17.1 C18.2 C19.2 C20.2 SL5.5 U$31.3 U$31.5 U$31.6 U$31.7
GND5: C21.1 C22.2 C23.2 C24.2 SL6.5 U$38.3 U$38.5 U$38.6 U$38.7
GND6: C25.1 C26.2 C27.2 C28.2 SL7.5 U$45.3 U$45.5 U$45.6 U$45.7
GND7: C29.1 C30.2 C31.2 C32.2 SL8.5 U$52.3 U$52.5 U$52.6 U$52.7
GND8: C33.1 C34.2 C35.2 C36.2 SL9.5 U$59.3 U$59.5 U$59.6 U$59.7
GND9: C37.1 C38.2 C39.2 C40.2 SL10.5 U$66.3 U$66.5 U$66.6 U$66.7
GND10: C41.1 C42.2 C43.2 C44.2 SL11.5 U$73.3 U$73.5 U$73.6 U$73.7
GND11: C45.1 C46.2 C47.2 C48.2 SL12.5 U$80.3 U$80.5 U$80.6 U$80.7
GND12: C49.1 C50.2 C51.2 C52.2 SL13.5 U$87.3 U$87.5 U$87.6 U$87.7
GND13: C53.1 C54.2 C55.2 C56.2 SL14.5 U$94.3 U$94.5 U$94.6 U$94.7
GND14: C57.1 C58.2 C59.2 C60.2 SL15.5 U$101.3 U$101.5 U$101.6 U$101.7
GND15: C61.1 C62.2 C63.2 C64.2 SL16.5 U$108.3 U$108.5 U$108.6 U$108.7
GND16: C65.1 C66.2 C67.2 C68.2 SL17.5 U$115.3 U$115.5 U$115.6 U$115.7
GND17: C69.1 C70.2 C71.2 C72.2 SL18.5 U$122.3 U$122.5 U$122.6 U$122.7
GND18: C73.1 C74.2 C75.2 C76.2 SL19.5 U$129.3 U$129.5 U$129.6 U$129.7
GND19: C77.1 C78.2 C79.2 C80.2 SL20.5 U$136.3 U$136.5 U$136.6 U$136.7
GND20: C81.1 C82.2 C83.2 C84.2 SL21.5 U$143.3 U$143.5 U$143.6 U$143.7
GND21: C85.1 C86.2 C87.2 C88.2 SL22.5 U$150.3 U$150.5 U$150.6 U$150.7
GND22: C89.1 C90.2 C91.2 C92.2 SL23.5 U$157.3 U$157.5 U$157.6 U$157.7
GND23: C93.1 C94.2 C95.2 C96.2 SL24.5 U$164.3 U$164.5 U$164.6 U$164.7
GND24: C97.1 C98.2 C99.2 C100.2 SL25.5 U$171.3 U$171.5 U$171.6 U$171.7
GND25: C101.1 C102.2 C103.2 C104.2 SL26.5 U$178.3 U$178.5 U$178.6 U$178.7
GND26: C105.1 C106.2 C107.2 C108.2 SL27.5 U$185.3 U$185.5 U$185.6 U$185.7
GND27: C109.1 C110.2 C111.2 C112.2 SL28.5 U$192.3 U$192.5 U$192.6 U$192.7
GND28: C113.1 C114.2 C115.2 C116.2 SL29.5 U$199.3 U$199.5 U$199.6 U$199.7
GND29: C117.1 C118.2 C119.2 C120.2 SL30.5 U$206.3 U$206.5 U$206.6 U$206.7
GND30: C121.1 C122.2 C123.2 C124.2 SL31.5 U$213.3 U$213.5 U$213.6 U$213.7
GND31: C125.1 C126.2 C127.2 C128.2 SL32.5 U$220.3 U$220.5 U$220.6 U$220.7
GND32: C129.1 C130.2 C131.2 C132.2 SL33.5 U$227.3 U$227.5 U$227.6 U$227.7
GND33: C133.1 C134.2 C135.2 C136.2 SL34.5 U$234.3 U$234.5 U$234.6 U$234.7
GND34: C137.1 C138.2 C139.2 C140.2 SL35.5 U$241.3 U$241.5 U$241.6 U$241.7
GND35: C141.1 C142.2 C143.2 C144.2 SL36.5 U$248.3 U$248.5 U$248.6 U$248.7
GND36: C145.1 C146.2 C147.2 C148.2 SL37.5 U$255.3 U$255.5 U$255.6 U$255.7
GND37: C149.1 C150.2 C151.2 C152.2 SL38.5 U$262.3 U$262.5 U$262.6 U$262.7
GND38: C153.1 C154.2 C155.2 C156.2 SL39.5 U$269.3 U$269.5 U$269.6 U$269.7
GND39: C157.1 C158.2 C159.2 C160.2 SL40.5 U$276.3 U$276.5 U$276.6 U$276.7
GND40: C161.1 C162.2 C163.2 C164.2 SL41.5 U$283.3 U$283.5 U$283.6 U$283.7
GND41: C165.1 C166.2 C167.2 C168.2 SL42.5 U$290.3 U$290.5 U$290.6 U$290.7
ST: SL1.1 U$4.2
ST1: SL2.1 U$10.2
ST2: SL3.1 U$17.2
ST3: SL4.1 U$24.2
ST4: SL5.1 U$31.2
ST5: SL6.1 U$38.2
ST6: SL7.1 U$45.2
ST7: SL8.1 U$52.2
ST8: SL9.1 U$59.2
ST9: SL10.1 U$66.2
ST10: SL11.1 U$73.2
ST11: SL12.1 U$80.2
ST12: SL13.1 U$87.2
ST13: SL14.1 U$94.2
ST14: SL15.1 U$101.2
ST15: SL16.1 U$108.2
ST16: SL17.1 U$115.2
ST17: SL18.1 U$122.2
ST18: SL19.1 U$129.2
ST19: SL20.1 U$136.2
ST20: SL21.1 U$143.2
ST21: SL22.1 U$150.2
ST22: SL23.1 U$157.2
ST23: SL24.1 U$164.2
ST24: SL25.1 U$171.2
ST25: SL26.1 U$178.2
ST26: SL27.1 U$185.2
ST27: SL28.1 U$192.2
ST28: SL29.1 U$199.2
ST29: SL30.1 U$206.2
ST30: SL31.1 U$213.2
ST31: SL32.1 U$220.2
ST32: SL33.1 U$227.2
ST33: SL34.1 U$234.2
ST34: SL35.1 U$241.2
ST35: SL36.1 U$248.2
ST36: SL37.1 U$255.2
ST37: SL38.1 U$262.2
ST38: SL39.1 U$269.2
ST39: SL40.1 U$276.2
ST40: SL41.1 U$283.2
ST41: SL42.1 U$290.2
VCC: C2.1 SL1.6 U$4.14 U$4.15
VCC1: C6.1 SL2.6 U$10.14 U$10.15
VCC2: C10.1 SL3.6 U$17.14 U$17.15
VCC3: C14.1 SL4.6 U$24.14 U$24.15
VCC4: C18.1 SL5.6 U$31.14 U$31.15
VCC5: C22.1 SL6.6 U$38.14 U$38.15
VCC6: C26.1 SL7.6 U$45.14 U$45.15
VCC7: C30.1 SL8.6 U$52.14 U$52.15
VCC8: C34.1 SL9.6 U$59.14 U$59.15
VCC9: C38.1 SL10.6 U$66.14 U$66.15
VCC10: C42.1 SL11.6 U$73.14 U$73.15
VCC11: C46.1 SL12.6 U$80.14 U$80.15
VCC12: C50.1 SL13.6 U$87.14 U$87.15
VCC13: C54.1 SL14.6 U$94.14 U$94.15
VCC14: C58.1 SL15.6 U$101.14 U$101.15
VCC15: C62.1 SL16.6 U$108.14 U$108.15
VCC16: C66.1 SL17.6 U$115.14 U$115.15
VCC17: C70.1 SL18.6 U$122.14 U$122.15
VCC18: C74.1 SL19.6 U$129.14 U$129.15
VCC19: C78.1 SL20.6 U$136.14 U$136.15
VCC20: C82.1 SL21.6 U$143.14 U$143.15
VCC21: C86.1 SL22.6 U$150.14 U$150.15
VCC22: C90.1 SL23.6 U$157.14 U$157.15
VCC23: C94.1 SL24.6 U$164.14 U$164.15
VCC24: C98.1 SL25.6 U$171.14 U$171.15
VCC25: C102.1 SL26.6 U$178.14 U$178.15
VCC26: C106.1 SL27.6 U$185.14 U$185.15
VCC27: C110.1 SL28.6 U$192.14 U$192.15
VCC28: C114.1 SL29.6 U$199.14 U$199.15
VCC29: C118.1 SL30.6 U$206.14 U$206.15
VCC30: C122.1 SL31.6 U$213.14 U$213.15
VCC31: C126.1 SL32.6 U$220.14 U$220.15
VCC32: C130.1 SL33.6 U$227.14 U$227.15
VCC33: C134.1 SL34.6 U$234.14 U$234.15
VCC34: C138.1 SL35.6 U$241.14 U$241.15
VCC35: C142.1 SL36.6 U$248.14 U$248.15
VCC36: C146.1 SL37.6 U$255.14 U$255.15
VCC37: C150.1 SL38.6 U$262.14 U$262.15
VCC38: C154.1 SL39.6 U$269.14 U$269.15
VCC39: C158.1 SL40.6 U$276.14 U$276.15
VCC40: C162.1 SL41.6 U$283.14 U$283.15
VCC41: C166.1 SL42.6 U$290.14 U$290.15
XOUT: C4.1 SL1.4 U$4.12
XOUT1: C8.1 SL2.4 U$10.12
XOUT2: C12.1 SL3.4 U$17.12
XOUT3: C16.1 SL4.4 U$24.12
XOUT4: C20.1 SL5.4 U$31.12
XOUT5: C24.1 SL6.4 U$38.12
XOUT6: C28.1 SL7.4 U$45.12
XOUT7: C32.1 SL8.4 U$52.12
XOUT8: C36.1 SL9.4 U$59.12
XOUT9: C40.1 SL10.4 U$66.12
XOUT10: C44.1 SL11.4 U$73.12
XOUT11: C48.1 SL12.4 U$80.12
XOUT12: C52.1 SL13.4 U$87.12
XOUT13: C56.1 SL14.4 U$94.12
XOUT14: C60.1 SL15.4 U$101.12
XOUT15: C64.1 SL16.4 U$108.12
XOUT16: C68.1 SL17.4 U$115.12
XOUT17: C72.1 SL18.4 U$122.12
XOUT18: C76.1 SL19.4 U$129.12
XOUT19: C80.1 SL20.4 U$136.12
XOUT20: C84.1 SL21.4 U$143.12
XOUT21: C88.1 SL22.4 U$150.12
XOUT22: C92.1 SL23.4 U$157.12
XOUT23: C96.1 SL24.4 U$164.12
XOUT24: C100.1 SL25.4 U$171.12
XOUT25: C104.1 SL26.4 U$178.12
XOUT26: C108.1 SL27.4 U$185.12
XOUT27: C112.1 SL28.4 U$192.12
XOUT28: C116.1 SL29.4 U$199.12
XOUT29: C120.1 SL30.4 U$206.12
XOUT30: C124.1 SL31.4 U$213.12
XOUT31: C128.1 SL32.4 U$220.12
XOUT32: C132.1 SL33.4 U$227.12
XOUT33: C136.1 SL34.4 U$234.12
XOUT34: C140.1 SL35.4 U$241.12
XOUT35: C144.1 SL36.4 U$248.12
XOUT36: C148.1 SL37.4 U$255.12
XOUT37: C152.1 SL38.4 U$262.12
XOUT38: C156.1 SL39.4 U$269.12
XOUT39: C160.1 SL40.4 U$276.12
XOUT40: C164.1 SL41.4 U$283.12
XOUT41: C168.1 SL42.4 U$290.12
YOUT: C3.1 SL1.3 U$4.10
YOUT1: C7.1 SL2.3 U$10.10
YOUT2: C11.1 SL3.3 U$17.10
YOUT3: C15.1 SL4.3 U$24.10
YOUT4: C19.1 SL5.3 U$31.10
YOUT5: C23.1 SL6.3 U$38.10
YOUT6: C27.1 SL7.3 U$45.10
YOUT7: C31.1 SL8.3 U$52.10
YOUT8: C35.1 SL9.3 U$59.10
YOUT9: C39.1 SL10.3 U$66.10
YOUT10: C43.1 SL11.3 U$73.10
YOUT11: C47.1 SL12.3 U$80.10
YOUT12: C51.1 SL13.3 U$87.10
YOUT13: C55.1 SL14.3 U$94.10
YOUT14: C59.1 SL15.3 U$101.10
YOUT15: C63.1 SL16.3 U$108.10
YOUT16: C67.1 SL17.3 U$115.10
YOUT17: C71.1 SL18.3 U$122.10
YOUT18: C75.1 SL19.3 U$129.10
YOUT19: C79.1 SL20.3 U$136.10
YOUT20: C83.1 SL21.3 U$143.10
YOUT21: C87.1 SL22.3 U$150.10
YOUT22: C91.1 SL23.3 U$157.10
YOUT23: C95.1 SL24.3 U$164.10
YOUT24: C99.1 SL25.3 U$171.10
YOUT25: C103.1 SL26.3 U$178.10
YOUT26: C107.1 SL27.3 U$185.10
YOUT27: C111.1 SL28.3 U$192.10
YOUT28: C115.1 SL29.3 U$199.10
YOUT29: C119.1 SL30.3 U$206.10
YOUT30: C123.1 SL31.3 U$213.10
YOUT31: C127.1 SL32.3 U$220.10
YOUT32: C131.1 SL33.3 U$227.10
YOUT33: C135.1 SL34.3 U$234.10
YOUT34: C139.1 SL35.3 U$241.10
YOUT35: C143.1 SL36.3 U$248.10
YOUT36: C147.1 SL37.3 U$255.10
YOUT37: C151.1 SL38.3 U$262.10
YOUT38: C155.1 SL39.3 U$269.10
YOUT39: C159.1 SL40.3 U$276.10
YOUT40: C163.1 SL41.3 U$283.10
YOUT41: C167.1 SL42.3 U$290.10
ZOUT: C1.2 SL1.2 U$4.8
ZOUT1: C5.2 SL2.2 U$10.8
ZOUT2: C9.2 SL3.2 U$17.8
ZOUT3: C13.2 SL4.2 U$24.8
ZOUT4: C17.2 SL5.2 U$31.8
ZOUT5: C21.2 SL6.2 U$38.8
ZOUT6: C25.2 SL7.2 U$45.8
ZOUT7: C29.2 SL8.2 U$52.8
ZOUT8: C33.2 SL9.2 U$59.8
ZOUT9: C37.2 SL10.2 U$66.8
ZOUT10: C41.2 SL11.2 U$73.8
ZOUT11: C45.2 SL12.2 U$80.8
ZOUT12: C49.2 SL13.2 U$87.8
ZOUT13: C53.2 SL14.2 U$94.8
ZOUT14: C57.2 SL15.2 U$101.8
ZOUT15: C61.2 SL16.2 U$108.8
ZOUT16: C65.2 SL17.2 U$115.8
ZOUT17: C69.2 SL18.2 U$122.8
ZOUT18: C73.2 SL19.2 U$129.8
ZOUT19: C77.2 SL20.2 U$136.8
ZOUT20: C81.2 SL21.2 U$143.8
ZOUT21: C85.2 SL22.2 U$150.8
ZOUT22: C89.2 SL23.2 U$157.8
ZOUT23: C93.2 SL24.2 U$164.8
ZOUT24: C97.2 SL25.2 U$171.8
ZOUT25: C101.2 SL26.2 U$178.8
ZOUT26: C105.2 SL27.2 U$185.8
ZOUT27: C109.2 SL28.2 U$192.8
ZOUT28: C113.2 SL29.2 U$199.8
ZOUT29: C117.2 SL30.2 U$206.8
ZOUT30: C121.2 SL31.2 U$213.8
ZOUT31: C125.2 SL32.2 U$220.8
ZOUT32: C129.2 SL33.2 U$227.8
ZOUT33: C133.2 SL34.2 U$234.8
ZOUT34: C137.2 SL35.2 U$241.8
ZOUT35: C141.2 SL36.2 U$248.8
ZOUT36: C145.2 SL37.2 U$255.8
ZOUT37: C149.2 SL38.2 U$262.8
ZOUT38: C153.2 SL39.2 U$269.8
ZOUT39: C157.2 SL40.2 U$276.8
ZOUT40: C161.2 SL41.2 U$283.8
ZOUT41: C165.2 SL42.2 U$290.8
